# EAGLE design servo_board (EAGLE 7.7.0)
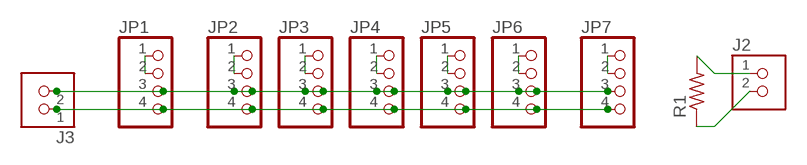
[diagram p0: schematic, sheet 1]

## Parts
J2  TERM-1X02-FABLAB  [ED555DS-2DS]
J3  TERM-1X02-ADAFRUIT  [3.5MMTERM]
JP1  PINHD-1X4  [1X04]
JP2  PINHD-1X4  [1X04]
JP3  PINHD-1X4  [1X04]
JP4  PINHD-1X4  [1X04]
JP5  PINHD-1X4  [1X04]
JP6  PINHD-1X4  [1X04]
JP7  PINHD-1X4  [1X04]
R1  RES-US1206  [R1206]

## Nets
N$2: J3.1 JP1.4 JP2.4 JP3.4 JP4.4 JP5.4 JP6.4 JP7.4
N$3: J2.1 R1.2
N$4: J2.2 R1.1
N$5: JP1.1 JP1.2
N$6: JP2.1 JP2.2
N$7: JP3.1 JP3.2
N$8: JP4.1 JP4.2
N$9: JP5.1 JP5.2
N$10: JP6.1 JP6.2
N$11: JP7.1 JP7.2
N$12: J3.2 JP1.3 JP2.3 JP3.3 JP4.3 JP5.3 JP6.3 JP7.3

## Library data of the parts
J2 J3 = fab:TERM-1X02: 3.5mm terminal block, 2 positions ED555-2DS as found in the fablab inventory.
JP1-JP7 = pinhead:PINHD-1X4: PIN HEADER
R1 = fab:RES-US: Resistor (US Symbol)

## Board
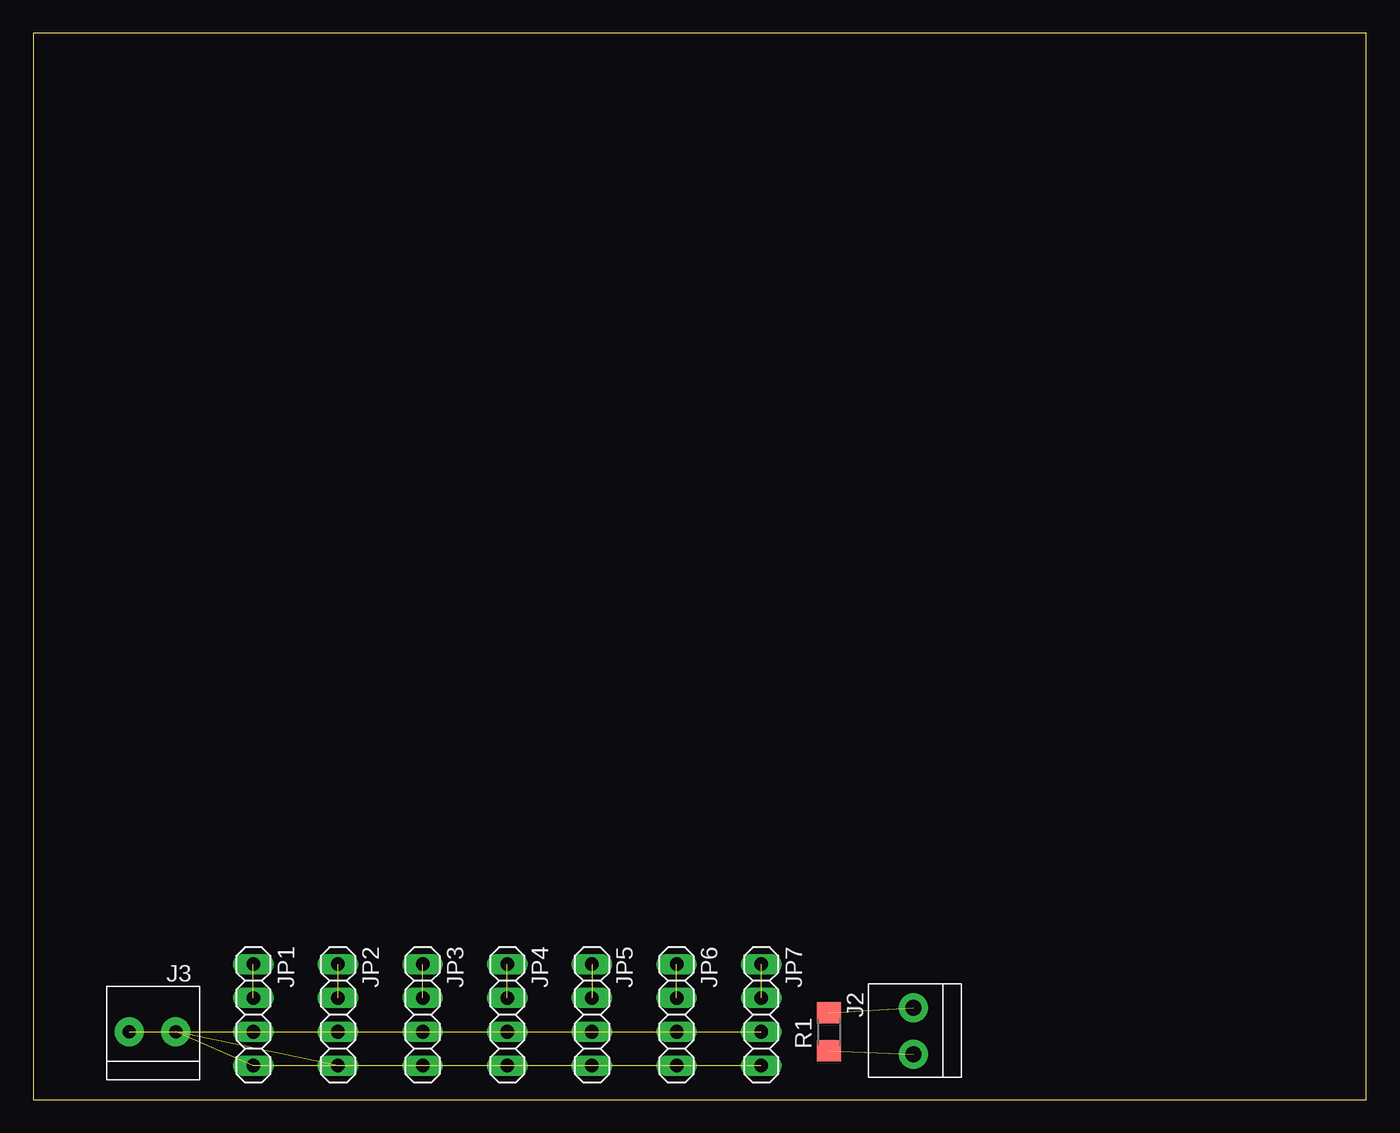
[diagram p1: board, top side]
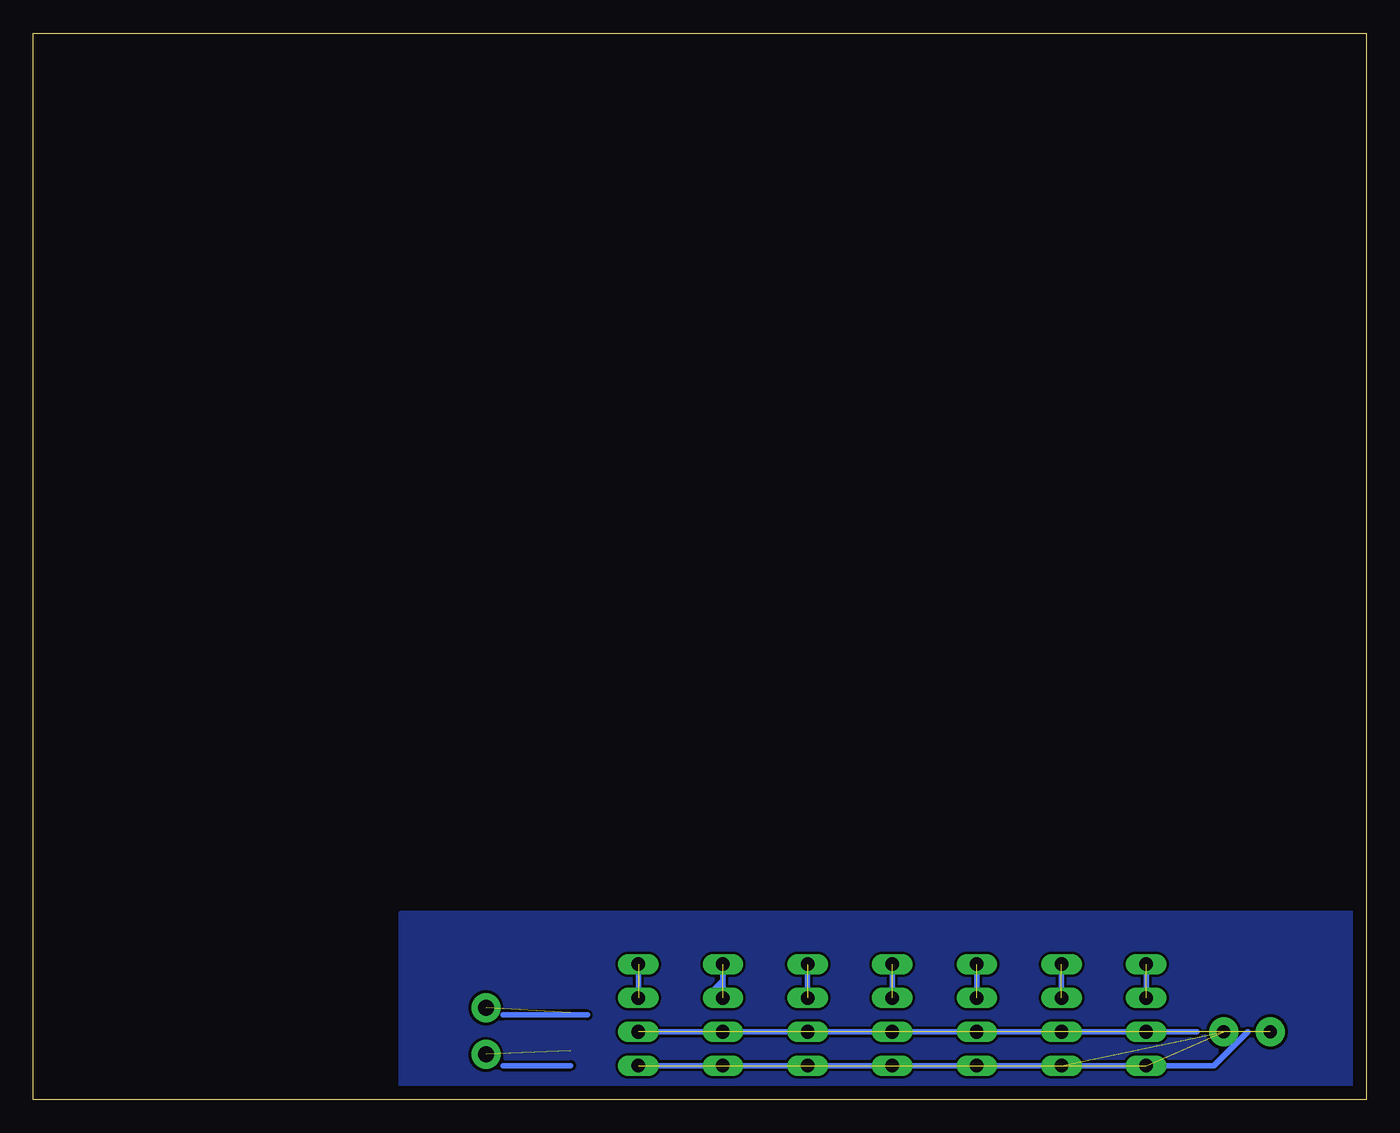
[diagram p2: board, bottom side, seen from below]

Size 100 x 80 mm. Coordinates in mm from the lower left corner, seen from the top.
Outline: 0,0 100,0 100,80 0,80 0,0
Copper layers (1*16): Top 0.035mm / dielectric 1.5mm / Bottom 0.035mm
Design rules "default": minimum track width 10mil, minimum drill 24mil, track to track 8mil, track to pad 8mil, pad to pad 8mil, via to via 8mil, smd to smd 8mil, copper to edge 40mil, drill to drill 8mil, minimum pad ring 10mil, minimum via ring 8mil, stop-mask expansion 4mil, vias tented up to drill 0mil, thermal gap 10mil

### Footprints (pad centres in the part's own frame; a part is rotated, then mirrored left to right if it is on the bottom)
ED555DS-2DS = drill 1.2 pad 2.184: 1 1.8,0; 2 -1.7,0
3.5MMTERM = drill 1 pad 2.184: 1 1.8,0; 2 -1.7,0
1X04 = drill 1.016 long: 1 -3.81,0; 2 -1.27,0; 3 1.27,0; 4 3.81,0
R1206 = smd 1.6 x 1.803: 1 -1.422,0; 2 1.422,0

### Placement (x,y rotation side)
J2  66.04,5.08 90 top
J3  8.89,5.08 0 top
JP1  16.51,6.35 270 top
JP2  22.86,6.35 270 top
JP3  29.21,6.35 270 top
JP4  35.56,6.35 270 top
JP5  41.91,6.35 270 top
JP6  48.26,6.35 270 top
JP7  54.61,6.35 270 top
R1  59.69,5.08 90 top

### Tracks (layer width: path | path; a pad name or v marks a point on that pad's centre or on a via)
N$1
  Bottom 0.406: 58.42,6.35 64.77,6.35
N$2  (7 unrouted)
  Bottom 0.406: 8.89,5.08 11.43,2.54 JP7.4 55.88,2.54
N$3  (1 unrouted)
N$4  (1 unrouted)
N$5  (1 unrouted)
  Bottom 0.406: JP1.2 JP1.1
N$6  (1 unrouted)
  Bottom 0.406: JP2.2 JP2.1
N$7  (1 unrouted)
  Bottom 0.406: JP3.2 JP3.1
N$8  (1 unrouted)
  Bottom 0.406: JP4.2 JP4.1
N$9  (1 unrouted)
  Bottom 0.406: JP5.2 JP5.1
N$10  (1 unrouted)
  Bottom 0.406: 49.53,7.62 48.26,8.89 JP6.1 JP6.2
N$11  (1 unrouted)
  Bottom 0.406: JP7.2 JP7.1
N$12  (7 unrouted)
  Bottom 0.406: JP7.3 12.7,5.08
N$13
  Bottom 0.406: 64.77,2.54 59.69,2.54
N$14
  pour Bottom: 0,13.97 72.39,13.97 72.39,0 0,0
